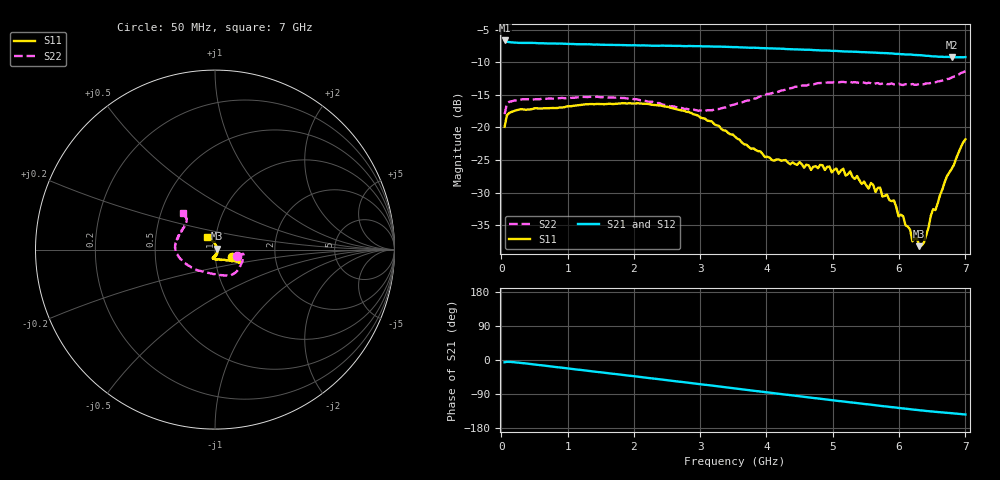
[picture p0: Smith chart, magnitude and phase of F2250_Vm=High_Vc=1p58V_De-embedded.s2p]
! Integrated Device Technology
! Corporate Headquarters
! 6024 Silver Creek Valley Road
! San Jose, CA 95138  USA
! Phone:  1-408-284-8200
! Toll Free:  1-800-223-1366
! Webpage:  http://www.idt.com/
! Timing and RF Division
! 515 Groton Road, Suite 102
! Westford, MA 01886-6024
! Device:  F2250
! Description: Voltage Variable RF Attenuator
! Frequency:  50.0 -  6000.00 MHz
! Package:  3x3 mm Thin QFN Plastic Package: 16 pin
! Ports:  2 RF, 3 DC
!  Pin  1  = GND
!  Pin  2  = NC
!  Pin  3  = RF1  = Port 1
!  Pin  4  = NC
!  Pin  5  = GND
!  Pin  6  = GND
!  Pin  7  = GND
!  Pin  8  = GND
!  Pin  9  = NC
!  Pin 10  = RF2  = Port 2
!  Pin 11  = NC
!  Pin 12  = GND
!  Pin 13  = GND
!  Pin 14  = VCNTRL
!  Pin 15  = VDD
!  Pin 16  = VMODE
! Vcntrl:  1.580 Volts
! Vmode:  +3.300 Volts
! Vdd:  +3.30  Volts
! Current:  1.328 mA
! Data:  The device was measured on a the F2250 evaluation board which has
!  individual transmission lines to the RF pins.  Data was collected
!  using a calibrated network analyzer.  The evaluation board was
!  de-embedded using a TRL calibration technique.
!  The reference plane is the edge of the package pin.
! Misc:  SN 10
!  Action Tracker AT0258
! Date Measured:  2014-11-26
! Date:  2015-10-15  MJV
! Note:
!  Integrated Device Technology supplies this data as a sample of measured
!  data at the package pin for this product.  Your particular data for this
!  product may vary.
!  Data was taken at 25 degrees C.
!  Integrated Device Technology reserves the right to change this data at anytime.
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# GHz S dB R 50
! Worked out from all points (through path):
!   201 points, 50 MHz to 7 GHz, reference 50 ohm
!   highest |S21| = -6.64 dB at 50 MHz (marker M1); lowest = -9.2 dB at 6.792 GHz (marker M2)
!   group delay of S21, straight-line fit = 57.6 ps
!   lowest |S11| = -38.2 dB at 6.305 GHz (marker M3), VSWR 1.02, Z = 51.2 + j0.448 ohm
!   |S11| at or under -10 dB: start of sweep to end of sweep
!   |S22| runs from -18.0 to -11.3 dB; largest |S21 - S12| = 0.0018
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0.05  -19.90 -23.1  -6.64 -6.0  -6.63 -6.0  -17.96 -17.2
0.08475  -18.12 -11.6  -6.83 -4.9  -6.83 -4.9  -16.36 -9.9
0.22375  -17.37 -8.3  -6.97 -6.4  -6.98 -6.4  -15.83 -10.8
1.2315  -16.48 -24.2  -7.22 -27.0  -7.21 -27.1  -15.31 -42.6
2.37825  -16.61 -28.0  -7.46 -50.5  -7.45 -50.6  -16.25 -70.9
2.969  -18.20 -30.6  -7.51 -63.1  -7.51 -63.1  -17.43 -97.5
3.525  -21.41 -43.7  -7.65 -75.0  -7.68 -75.1  -16.46 -130.6
4.081  -25.00 -71.7  -7.86 -87.0  -7.85 -87.0  -14.75 -156.1
4.7065  -26.04 -101.1  -8.11 -100.1  -8.12 -100.1  -13.37 -174.5
5.2625  -26.74 -97.2  -8.34 -111.6  -8.37 -111.6  -13.01 172.5
5.85325  -31.18 -72.4  -8.62 -123.6  -8.61 -123.8  -13.34 156.3
5.92275  -31.22 -68.6  -8.67 -125.0  -8.67 -125.0  -13.39 155.5
5.99225  -33.66 -63.1  -8.70 -126.5  -8.69 -126.6  -13.28 153.0
6.166  -35.71 -31.8  -8.79 -129.9  -8.82 -129.9  -13.44 146.8
6.20075  -37.50 -22.2  -8.83 -130.6  -8.85 -130.6  -13.32 146.2
6.27025  -37.06 -2.1  -8.88 -131.9  -8.88 -131.9  -13.44 143.5
6.305  -38.24 20.9  -8.89 -132.6  -8.91 -132.6  -13.30 142.6
6.3745  -37.67 37.4  -8.95 -133.9  -8.96 -133.9  -13.37 139.9
6.5135  -32.54 77.5  -9.08 -136.1  -9.08 -136.3  -13.10 136.4
6.54825  -32.70 85.0  -9.07 -136.8  -9.08 -136.9  -13.06 135.8
6.7915  -26.39 106.0  -9.22 -140.3  -9.21 -140.5  -12.34 131.8
7  -21.82 121.4  -9.19 -143.8  -9.21 -143.9  -11.35 131.3
